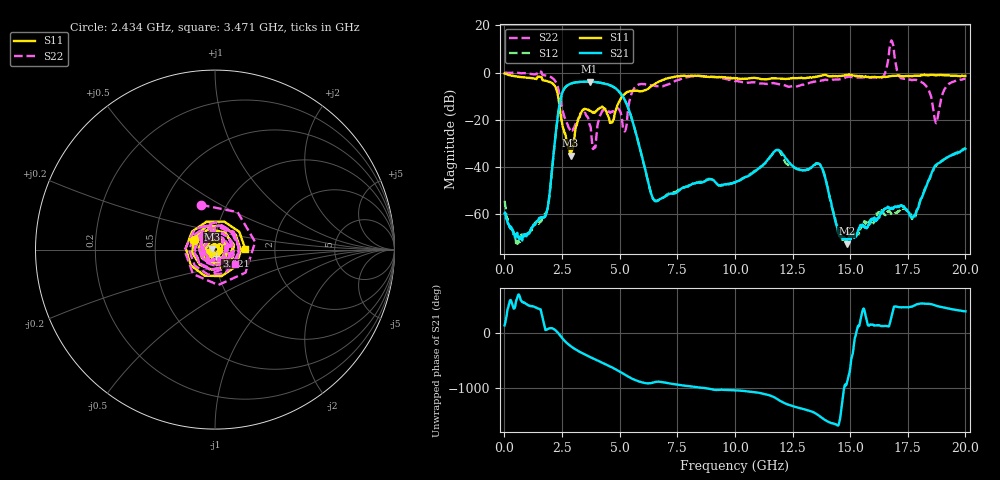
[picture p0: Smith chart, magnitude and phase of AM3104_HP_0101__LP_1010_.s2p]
!Created with skrf (http://scikit-rf.org).
# Hz S RI R 50.0
!freq ReS11 ImS11 ReS21 ImS21 ReS12 ImS12 ReS22 ImS22
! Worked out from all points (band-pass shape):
!   1601 points, 10 MHz to 20 GHz, reference 50 ohm
!   highest |S21| = -3.80 dB at 3.696 GHz (marker M1); lowest = -72.5 dB at 14.85 GHz (marker M2)
!   |S21| within 3 dB of the highest: 2.598 GHz to 4.842 GHz (2.244 GHz wide, 60.3 % of centre)
!   lowest |S11| = -35.3 dB at 2.871 GHz (marker M3), VSWR 1.04, Z = 48.3 + j0.268 ohm
!   |S11| at or under -10 dB: 2.328 GHz to 5.129 GHz (2.801 GHz wide, 75.1 % of centre)
!   |S22| runs from -32.4 to 13.6 dB; largest |S21 - S12| = 0.052
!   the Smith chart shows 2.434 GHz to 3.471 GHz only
!   S11 on the Smith chart (normalised r, x): 2.434 GHz: 0.78, +0.09; 3.021 GHz: 1.01, -0.07; 3.471 GHz: 1.41, +0.00
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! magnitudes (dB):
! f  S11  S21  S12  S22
! 10 MHz  -0.4  -59.6  -54.4  0.0
! 584.7 MHz  -1.7  -69.8  -72.3  -0.1
! 1.797 GHz  -3.5  -60.6  -59.6  -1.2
! 2.434 GHz  -17.7  -11.3  -11.4  -11.6
! 2.871 GHz  -35.3  -4.7  -4.8  -24.7
! 3.021 GHz  -29.2  -4.3  -4.3  -23.4
! 3.346 GHz  -16.7  -3.9  -4.0  -17.2
! 3.471 GHz  -15.4  -3.9  -3.9  -17.1
! 3.696 GHz  -16.1  -3.8  -3.9  -22.1
! 3.896 GHz  -16.7  -3.9  -3.9  -31.5
! 4.658 GHz  -21.1  -5.6  -5.8  -16.6
! 5.17 GHz  -9.5  -10.6  -10.7  -24.3
! 5.682 GHz  -7.6  -24.8  -24.9  -6.0
! 6.682 GHz  -4.0  -54.1  -54.3  -5.8
! 10.01 GHz  -2.5  -46.8  -46.6  -3.6
! 11.83 GHz  -2.5  -32.9  -32.9  -4.8
! 13.34 GHz  -2.1  -40.1  -40.1  -4.1
! 14.85 GHz  -1.0  -72.5  -68.1  -2.0
! 16.68 GHz  -1.6  -57.6  -58.6  7.3
! 17.74 GHz  -1.4  -61.0  -61.8  -3.1
! 18.73 GHz  -1.2  -39.1  -39.5  -21.4
! 20 GHz  -1.4  -32.4  -32.1  -2.6
